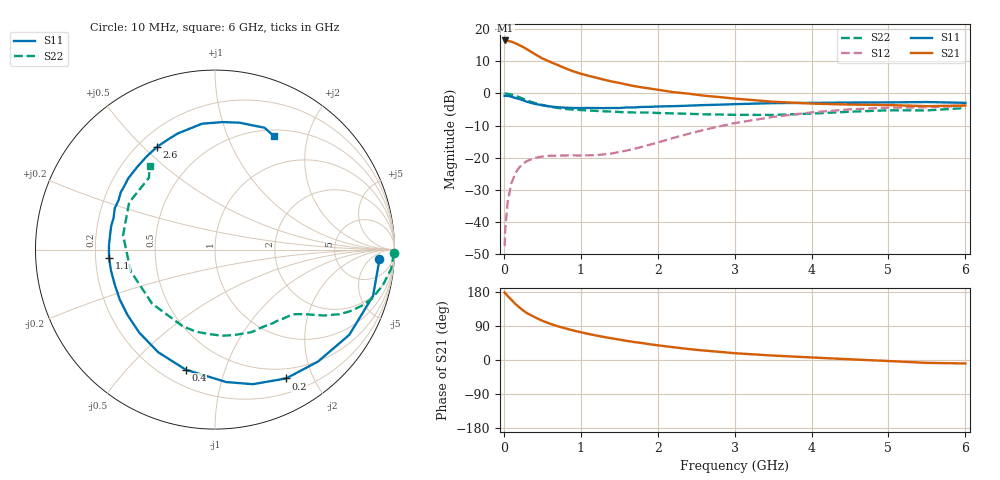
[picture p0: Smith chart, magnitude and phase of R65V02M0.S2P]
! SIEMENS Small Signal Semiconductors
! BFR193
! Si NPN RF Bipolar Junction Transistor in SOT23
! VCE = 5 V  IC = 2 mA
! Common Emitter S-Parameters:  May  1996
# GHz  S  MA  R  50
!  f  S11  S21  S12  S22
! GHz  MAG  ANG  MAG  ANG  MAG  ANG  MAG  ANG
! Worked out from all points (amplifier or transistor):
!   36 points, 10 MHz to 6 GHz, reference 50 ohm
!   highest |S21| = 16.5 dB at 20 MHz (marker M1)
!   |S21| within 3 dB of that: start of sweep to 318.3 MHz
!   unconditionally stable (mu >= 1): 1.168 GHz to 2.011 GHz
!   at 250 MHz: K = 0.23, MSG = 18.1 dB, |S12| = -21.8 dB
!   at 1.4 GHz: K = 1.11, MAG = 9.2 dB, |S12| = -18.7 dB
!   at 6 GHz: K = 0.99, MSG = 0.1 dB, |S12| = -3.9 dB
!   S11 on the Smith chart (normalised r, x): 10 MHz: 16, -11; 200 MHz: 0.37, -1.63; 400 MHz: 0.29, -0.74; 1.1 GHz: 0.26, -0.04; 2.6 GHz: 0.27, +0.55; 6 GHz: 0.58, +1.49
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0.01  0.9176 -3.4  6.612 178.1  0.0042 86.9  0.9984 -1.2
0.02  0.9136 -6.6  6.654 175.5  0.0081 85.6  0.9937 -2.5
0.05  0.9176 -16.3  6.548 169.0  0.0209 80.6  0.9867 -6.3
0.1  0.8861 -32.4  6.37 158.5  0.0406 72.3  0.9558 -12.0
0.15  0.8476 -47.4  6.024 147.9  0.0571 64.0  0.9156 -17.4
0.2  0.8199 -61.1  5.629 139.2  0.0706 58.0  0.8722 -21.2
0.25  0.779 -74.3  5.258 130.9  0.0809 52.1  0.8247 -24.7
0.3  0.7404 -85.2  4.86 123.8  0.0886 47.9  0.7799 -27.5
0.4  0.6886 -103.7  4.099 113.2  0.0989 41.0  0.7108 -31.1
0.5  0.6534 -119.0  3.5 103.6  0.1042 36.6  0.6606 -33.4
0.6  0.6261 -132.4  3.099 95.7  0.1073 34.1  0.6221 -35.4
0.7  0.6088 -143.0  2.759 89.1  0.1075 33.1  0.5933 -37.3
0.9  0.5918 -160.5  2.207 78.1  0.1086 33.7  0.5592 -40.7
1.1  0.5924 -175.4  1.879 68.8  0.1086 37.5  0.5417 -45.0
1.4  0.593 167.4  1.532 57.2  0.1162 47.7  0.5212 -52.1
1.6  0.6042 157.6  1.369 50.3  0.1291 54.3  0.5078 -57.5
2.2  0.6322 133.4  1.046 33.8  0.202 64.1  0.4882 -77.0
2.6  0.6575 119.3  0.921 25.0  0.2701 62.4  0.4723 -93.5
3.5  0.7051 95.9  0.741 11.7  0.4302 47.4  0.4621 -139.3
4.5  0.7202 79.1  0.669 1.9  0.5639 26.4  0.5184 171.1
5.5  0.7329 67.9  0.632 -7.6  0.6068 7.0  0.5438 132.6
6  0.7129 62.6  0.648 -9.1  0.6404 1.7  0.5913 128.1
